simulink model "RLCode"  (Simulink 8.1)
settings: Solver=ode23t  StartTime=0.0  StopTime=100  RelTol=1e-3
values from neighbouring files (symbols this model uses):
  U = 5    [MotorDCParam.m]
undefined symbols (not defined in the file or in its folder): C, L, R

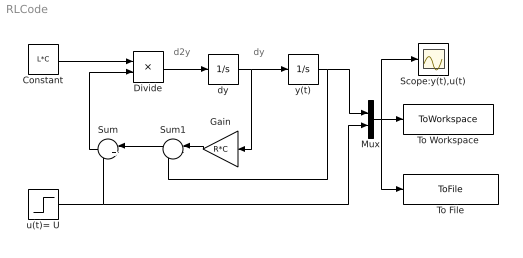
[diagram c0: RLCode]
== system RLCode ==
  note: dy
  note: d2y
  Constant : Constant  Value=L*C
  Divide : Product  Inputs=/*
  Gain : Gain  Gain=R*C
  Mux : Mux  Inputs=2
  Scope:y(t),u(t) : Scope
  Sum : Sum  Inputs=|++
  Sum1 : Sum  Inputs=|--
  To File : ToFile  Filename=RLCOde.mat  SaveFormat=Timeseries
  To Workspace : ToWorkspace  VariableName=RLCOde  SampleTime=-1
  dy : Integrator
  u(t)= U : Step  Time=0  After=U  SampleTime=0
  y(t) : Integrator
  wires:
  u(t)= U/1 -> Mux/2, Sum/2
  Mux/1 -> To File/1, To Workspace/1, Scope:y(t),u(t)/1
  dy/1 -> Gain/1, y(t)/1
  Gain/1 -> Sum1/1
  y(t)/1 -> Sum1/2, Mux/1
  Sum1/1 -> Sum/1
  Divide/1 -> dy/1
  Constant/1 -> Divide/1
  Sum/1 -> Divide/2
